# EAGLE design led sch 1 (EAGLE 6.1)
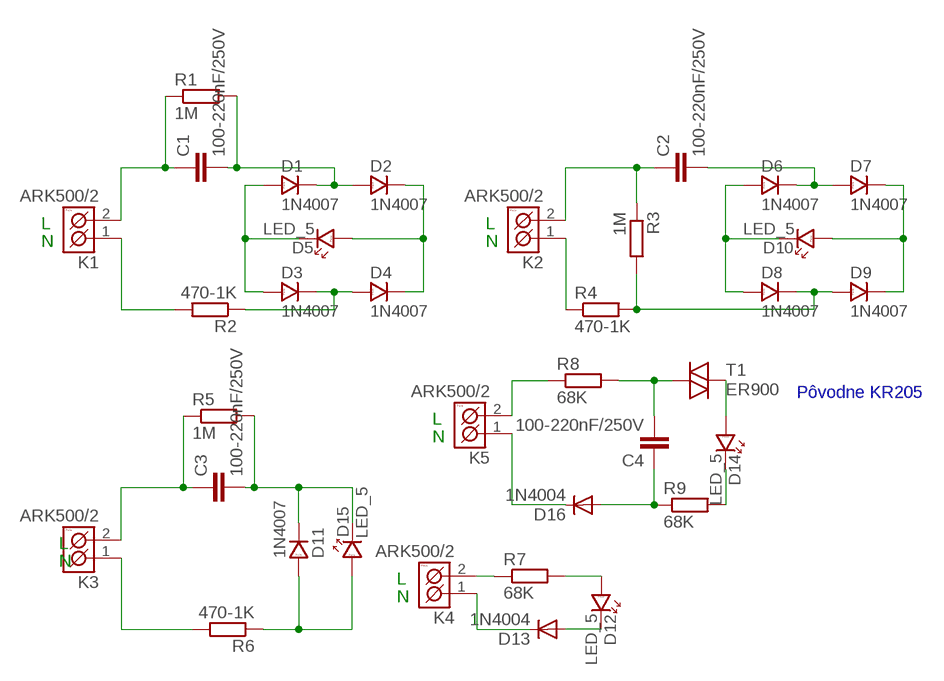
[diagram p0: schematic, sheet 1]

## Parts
C1  100-220nF/250V  FOLIOVYRM10/5-13  [FOLIOVY_RM10/5-13]
C2  100-220nF/250V  FOLIOVYRM10/5-13  [FOLIOVY_RM10/5-13]
C3  100-220nF/250V  FOLIOVYRM10/5-13  [FOLIOVY_RM10/5-13]
C4  100-220nF/250V  FOLIOVYRM10/5-13  [FOLIOVY_RM10/5-13]
D1  1N4007  1N4007_10  [DO41]
D2  1N4007  1N4007_10  [DO41]
D3  1N4007  1N4007_10  [DO41]
D4  1N4007  1N4007_10  [DO41]
D5  LED_5  [LED_5]
D6  1N4007  1N4007_10  [DO41]
D7  1N4007  1N4007_10  [DO41]
D8  1N4007  1N4007_10  [DO41]
D9  1N4007  1N4007_10  [DO41]
D10  LED_5  [LED_5]
D11  1N4007  1N4007_10  [DO41]
D12  LED_5  [LED_5]
D13  1N4004  [DO41-10]
D14  LED_5  [LED_5]
D15  LED_5  [LED_5]
D16  1N4004  [DO41-10]
K1  ARK500/2  [ARK500/2]
K2  ARK500/2  [ARK500/2]
K3  ARK500/2  [ARK500/2]
K4  ARK500/2  [ARK500/2]
K5  ARK500/2  [ARK500/2]
R1  1M  R-EU_0207/7  [0207/7]
R2  470-1K  R-EU_0207/7  [0207/7]
R3  1M  R-EU_0207/7  [0207/7]
R4  470-1K  R-EU_0207/7  [0207/7]
R5  1M  R-EU_0207/7  [0207/7]
R6  470-1K  R-EU_0207/7  [0207/7]
R7  68K  R-EU_0207/7  [0207/7]
R8  68K  R-EU_0207/7  [0207/7]
R9  68K  R-EU_0207/7  [0207/7]
T1  ER900  [ER900]

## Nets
N$1: D1.A D3.A D5.K
N$2: C1.P$2 D1.K D2.A R1.2
N$3: D2.K D4.K D5.A
N$4: D3.K D4.A R2.1
N$5: C1.P$1 K1.2(K2) R1.1
N$6: K1.1(K1) R2.2
N$7: D6.A D8.A D10.K
N$8: C2.P$2 D6.K D7.A
N$9: D7.K D9.K D10.A
N$10: K2.1(K1) R4.1
N$11: C2.P$1 K2.2(K2) R3.1
N$12: D8.K D9.A R3.2 R4.2
N$13: K4.2(K2) R7.1
N$14: C3.P$2 D11.K D15.K R5.2
N$15: D13.C K4.1(K1)
N$16: D11.A D15.A R6.1
N$17: C3.P$1 K3.2(K2) R5.1
N$18: K3.1(K1) R6.2
N$19: D12.A R7.2
N$20: D12.K D13.A
N$21: K5.2(K2) R8.1
N$22: D16.C K5.1(K1)
N$23: C4.P$2 R8.2 T1.1
N$24: D14.A T1.2
N$25: D14.K R9.2
N$26: C4.P$1 D16.A R9.1

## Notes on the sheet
- L | L
- N | N
- Pôvodne KR205
- L
- N
- L
- N
- L
- N

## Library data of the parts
C1-C4 = #Kondenzatory:FOLIOVY
D1-D4 D6-D9 D11 = #PaJa_30:1N4007: Usmernovaci dioda - 1A, 1000V
D5 D10 D12 D14 D15 = #PaJa_30:LED: LED - jednobarevna
D13 D16 = diode:1N4004: DIODE
K1-K5 = #PaJa_konektory:ARK500/2: Svorkovnice - roztec 5mm - dvojita
R1-R9 = #Odpory:R-EU_: RESISTOR, European symbol
T1 = triac:ER900: TRIGGER DIODE

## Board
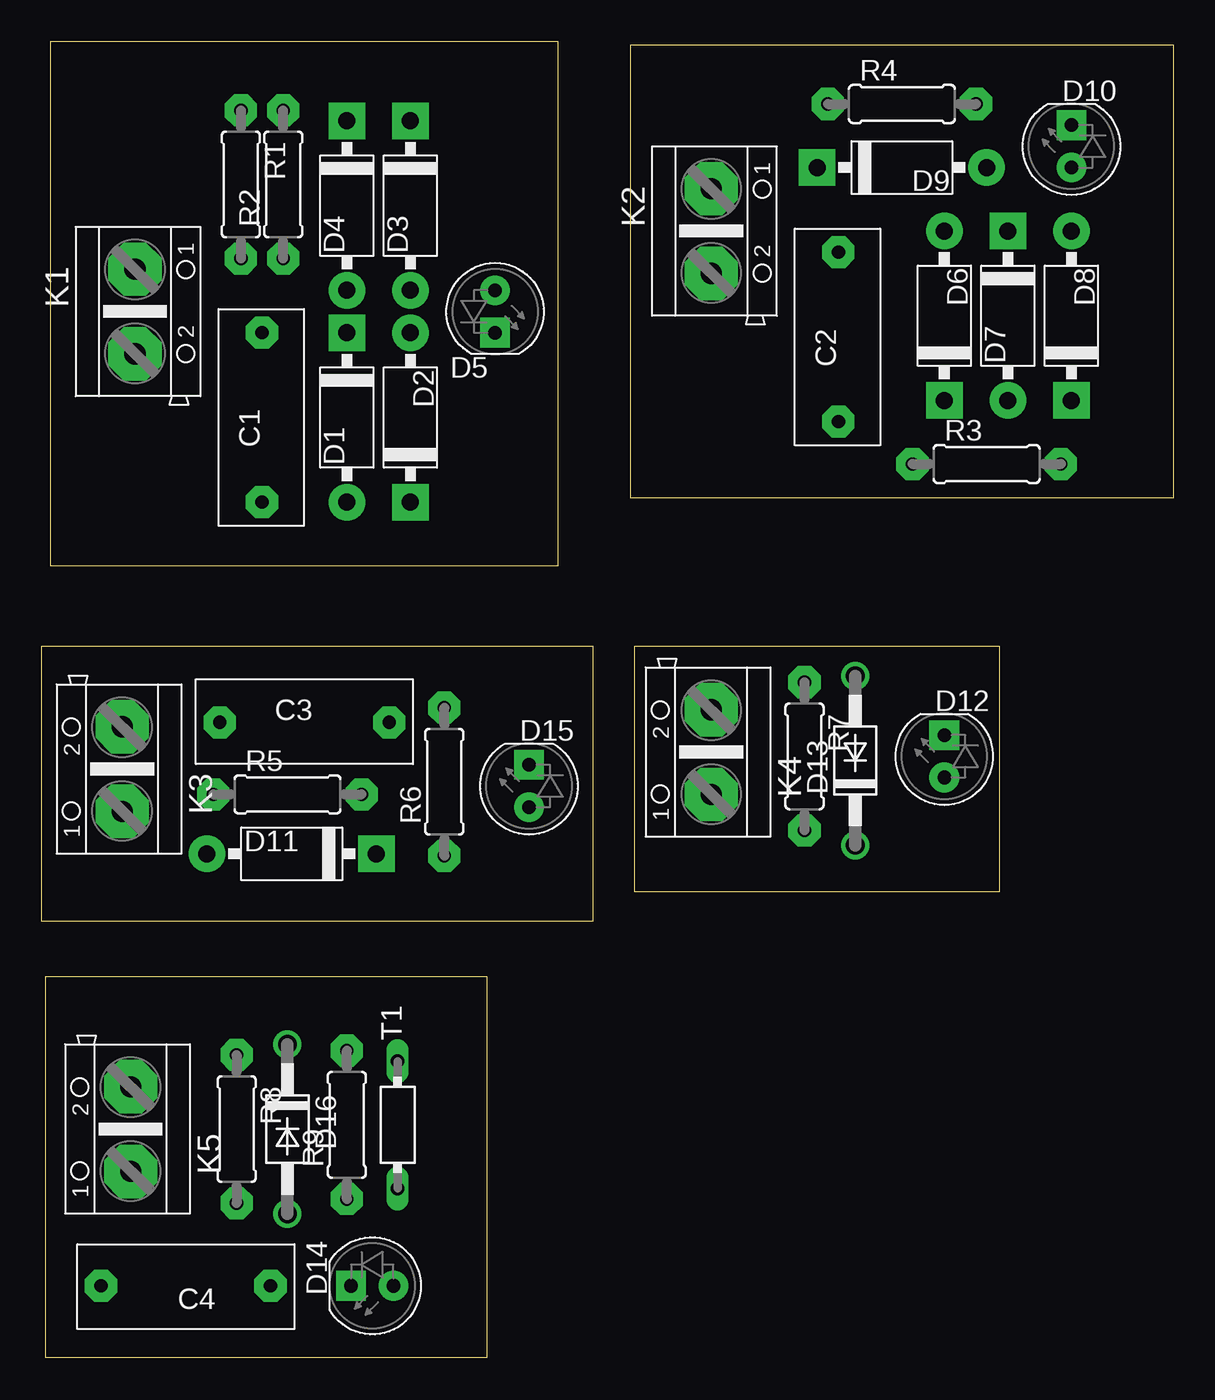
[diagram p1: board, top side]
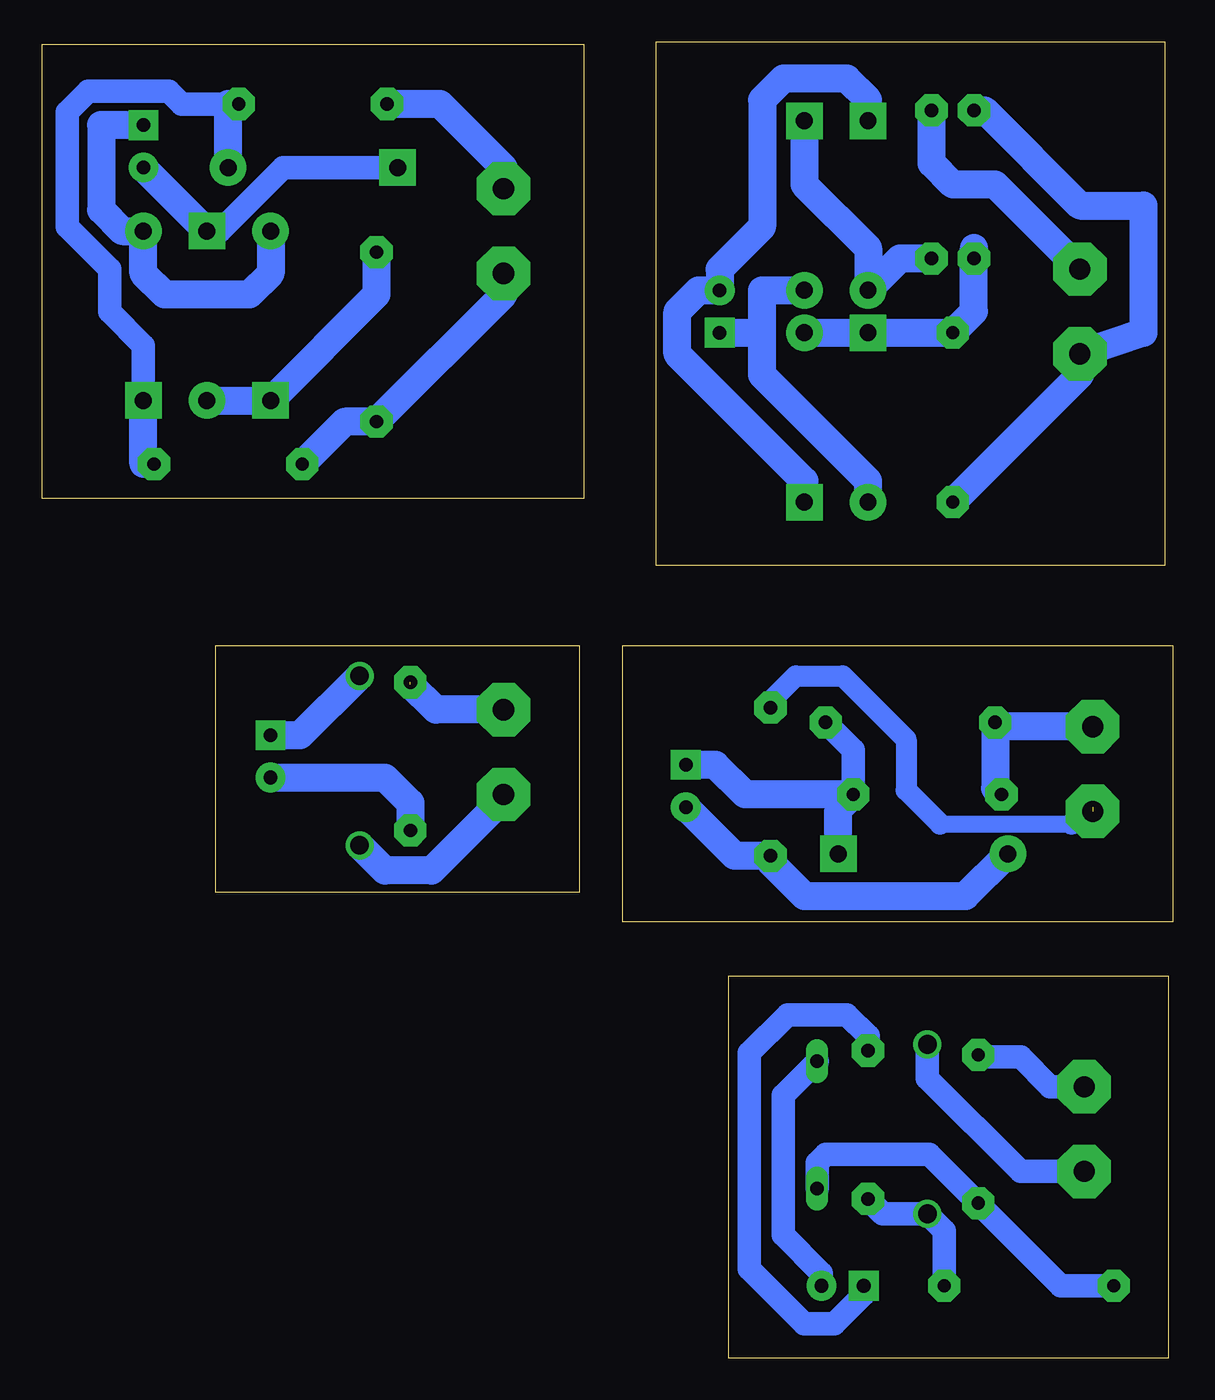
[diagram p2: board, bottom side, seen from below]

Size 67.82 x 78.92 mm. Coordinates in mm from the lower left corner, seen from the top.
Outline: 0.51,47.5 30.97,47.5 30.97,78.92 0.51,78.92 0.51,47.5
Outline: 35.31,78.74 67.82,78.74 67.82,51.56 35.31,51.56 35.31,78.74
Outline: 0,42.67 33.02,42.67 33.02,26.16 0,26.16 0,42.67
Outline: 35.56,42.67 57.4,42.67 57.4,27.94 35.56,27.94 35.56,42.67
Outline: 0.25,22.86 26.67,22.86 26.67,0 0.25,0 0.25,22.86
Copper layers (1*16): Top 0.035mm / dielectric 1.5mm / Bottom 0.035mm
Design rules: minimum track width 10mil, minimum drill 24mil, track to track 8mil, track to pad 8mil, pad to pad 8mil, via to via 8mil, smd to smd 8mil, copper to edge 40mil, drill to drill 8mil, minimum pad ring 10mil, minimum via ring 8mil, stop-mask expansion 4mil, vias tented up to drill 0mil, thermal gap 10mil

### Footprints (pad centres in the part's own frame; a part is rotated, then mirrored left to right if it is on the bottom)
FOLIOVY_RM10/5-13 = drill 0.8 pad 1.93 octagon: P$1 -5.08,0; P$2 5.08,0
DO41 = drill 1.016 pad 2.184: A -5.08,0 | drill 1.016 pad 2.184 square: K 5.08,0
LED_5 = drill 0.813 pad 1.778: A -1.27,0 | drill 0.813 pad 1.778 square: K 1.27,0
DO41-10 = drill 1.118: A 5.08,0; C -5.08,0
ARK500/2 = drill 1.27 pad 3.2 octagon: 1 -2.54,0; 2 2.54,0
0207/7 = drill 0.8 pad 1.93 octagon: 1 -4.445,0; 2 4.445,0
ER900 = drill 0.813 long: 1 -3.81,0; 2 3.81,0

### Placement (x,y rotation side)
C1  13.21,56.39 90 top
C2  47.75,61.21 90 top
C3  15.75,38.1 0 top
C4  8.64,4.32 180 top
D1  18.29,56.39 90 top
D2  22.1,56.39 270 top
D3  22.1,69.09 90 top
D4  18.29,69.09 90 top
D5  27.18,62.74 270 top
D6  54.1,62.48 270 top
D7  57.91,62.48 90 top
D8  61.72,62.48 270 top
D9  51.56,71.37 180 top
D10  61.72,72.64 90 top
D11  14.99,30.23 0 top
D12  54.1,36.07 90 top
D13  48.77,35.81 90 top
D14  19.81,4.32 180 top
D15  29.21,34.29 90 top
D16  14.73,13.72 270 top
K1  5.59,62.74 270 top
K2  40.13,67.56 270 top
K3  4.83,35.31 90 top
K4  40.13,36.32 90 top
K5  5.33,13.72 90 top
R1  11.94,70.36 270 top
R2  14.48,70.36 90 top
R3  56.64,53.59 0 top
R4  51.56,75.18 0 top
R5  14.73,33.78 0 top
R6  24.13,34.54 90 top
R7  45.72,36.07 270 top
R8  11.68,13.72 270 top
R9  18.29,13.97 90 top
T1  21.34,13.97 90 top

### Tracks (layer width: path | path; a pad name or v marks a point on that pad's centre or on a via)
N$1
  Bottom 1.676: D1.A 18.29,52.58 24.64,58.93 24.64,61.47 | 24.64,61.47 24.64,64.01 D3.A | D5.K 24.64,61.47
N$2
  Bottom 1.676: 11.94,66.55 R1.2 11.94,62.74 C1.P$2 D1.K D2.A
N$3
  Bottom 1.676: D4.K 18.29,75.44 19.56,76.71 23.37,76.71 24.64,75.44 24.64,67.82 27.18,65.28 D5.A 28.45,64.01 29.72,62.74 29.72,60.2 22.1,52.58 D2.K
N$4
  Bottom 1.676: D3.K 22.1,70.36 18.29,66.55 D4.A 16.38,65.91 R2.1
N$5
  Bottom 1.676: C1.P$1 5.59,58.93 K1.2 1.78,61.47 1.78,69.09 5.59,69.09 11.3,74.8 R1.1
N$6
  Bottom 1.676: K1.1 10.67,70.36 13.21,70.36 14.48,71.63 R2.2
N$7
  Bottom 1.676: D6.A 54.1,65.02 55.37,63.75 60.45,63.75 61.72,65.02 D8.A 62.99,67.56 64.26,68.83 64.26,73.91 D10.K
N$8
  Bottom 1.676: D7.A D6.K 47.75,63.75 C2.P$2
N$9
  Bottom 1.422: D7.K 57.15,67.56 53.34,71.37 D9.K
  Bottom 1.676: D10.A D7.K
N$10
  Bottom 1.676: K2.1 40.13,71.37 43.94,75.18 R4.1
N$11
  Bottom 1.676: K2.2 40.13,63.75 C2.P$1 49.66,56.13 R3.1
N$12
  Bottom 1.422: 56.64,75.18 59.44,75.18 60.2,75.95 65.02,75.95 66.29,74.68 66.29,67.82 63.75,65.28 63.75,62.74 61.72,60.71 D8.K
  Bottom 1.676: R3.2 61.72,53.59 D8.K | D9.A 56.64,74.55 R4.2 56.64,75.18
N$13  (1 unrouted)
  Bottom 1.676: K4.2 44.2,38.86 45.72,40.39
N$14
  Bottom 1.422: R5.2 19.18,36.45 C3.P$2
  Bottom 1.676: D11.K 20.07,32.89 R5.2 25.65,33.78 27.43,35.56 D15.K
N$15
  Bottom 1.676: K4.1 40.13,33.53 44.45,29.21 47.24,29.21 D13.C
N$16
  Bottom 1.676: D15.A 26.29,30.1 R6.1 24.13,29.72 22.1,27.69 12.45,27.69 D11.A
N$17
  Bottom 1.676: K3.2 10.41,37.85 C3.P$1 10.67,34.16 R5.1
N$18  (1 unrouted)
  Bottom 1.016: 13.97,32 6.1,32
  Bottom 1.27: R6.2 24.13,39.37 22.61,40.89 19.81,40.89 16,37.08 16,34.04 13.97,32 | 6.1,32 4.83,33.02
  Bottom 1.676: K3.1 4.57,32.77
N$19
  Bottom 1.676: D12.A 47.24,34.8 45.72,33.27 R7.2
N$20
  Bottom 1.676: D12.K 52.32,37.34 D13.A
N$21
  Bottom 1.422: K5.2 7.37,16.26 9.14,18.03 11.56,18.03 R8.1
N$22
  Bottom 1.422: K5.1 9.14,11.18 14.73,16.76 D16.C
N$23
  Bottom 1.422: 3.3,4.32 C4.P$2 6.73,4.32 R8.2 14.61,12.19 20.83,12.19 21.34,11.68 T1.1
N$24
  Bottom 1.422: D14.A 21.08,5.08 23.37,7.37 23.37,15.75 T1.2
N$25
  Bottom 1.422: D14.K 18.54,3.81 20.32,2.03 22.1,2.03 25.4,5.33 25.4,18.29 23.11,20.57 19.56,20.57 18.29,19.3 R9.2
N$26
  Bottom 1.422: C4.P$1 13.72,7.62 D16.A 17.4,8.64 R9.1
